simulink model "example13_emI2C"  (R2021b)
settings: Solver=FixedStepAuto  StartTime=0  StopTime=inf  FixedStep=0.5  RelTol=1e-3  EnableMultiTasking=on
undefined symbols (not defined in the file or in its folder): based, Big, bits, bus, classic, dsPic33, Endian, I2C, MCC, Microchip, PIC24
libraries: emSPII2CLib x6, embeddedCreatorLib x6, emMBSlaveLib x1

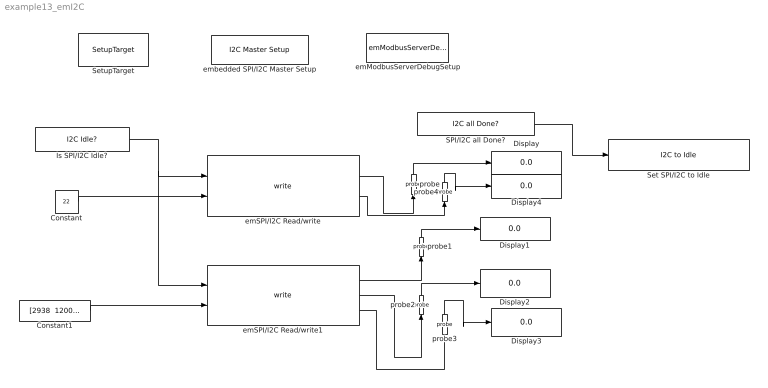
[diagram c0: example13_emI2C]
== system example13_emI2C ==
  Constant : Constant  Value=22  OutDataTypeStr=int8
  Constant1 : Constant  Value="[2938  12000]"  OutDataTypeStr=int16
  Display{,1..4} (5 alike) : Display
  Is SPI/I2C Idle? : emSPII2CLib/Is SPI//I2C Idle?  Tag=isSPI_I2C_Idle  c_DeviceNo=2  c_BusType=I2C bus  c_sampleTime=-1
  SPI/I2C all Done? : emSPII2CLib/SPI//I2C all Done?  c_DeviceNo=2  c_BusType=I2C bus  c_sampleTime=-1
  Set SPI/I2C to Idle : emSPII2CLib/Set SPI//I2C to Idle  Tag=setSPI_I2C2Idle  c_DeviceNo=2  c_BusType=I2C bus
  SetupTarget : embeddedCreatorLib/SetupTarget  Tag=SetupTarget  Priority=0  c_platform=Microchip PIC24/dsPic33 based on MCC classic  c_debug=on
  emModbusServerDebugSetup : emMBSlaveLib/emModbusServerDebugSetup  Tag=emModbusSlaveSetup  c_objID=0  c_uartNo=2  c_baudrate=19200  c_serverID=1  c_baudrate4PC=19200  c_forceLongerSpace=on  c_holdingRegsQTY=0  c_minHoldingAddr=789  c_inputRegsQTY=0  c_minInputRegAddr=20  c_coilRegsQTY=0  c_minCoilAddr=30  c_discreteRegsQTY=0  c_minDiscreteAddr=40  c_enableDebug=on  c_breakpointMaxQTY=0  c_probeMaxWordQTY=100  c_emWaitQTY=0  g_COMPortNo=COM5  c_Name_method=By physical port name and bit number  c_PortName=B  c_BitNo=11  c_TxEnable485="\"LATBbits.LATB11\""  c_TxEnable485Polarity=on
  emSPI/I2C Read/write : emSPII2CLib/emSPI//I2C Read//write  Tag=emSPII2CWR  c_DeviceNo=2  c_BusType=I2C bus  c_SeqNo=Seq0  c_How_to_specifyCS=By physical port name and bit number  c_PortName=D  c_BitNumber=8  c_CSAccessName="\"LATDbits.LATD8\""  c_CS_Polarity=on  c_SPI_dummyData=ALL bits Logic low  c_I2CAddress=1  c_Endian=Big-Endian  c_WriteDataType=[int8]  c_InputDataQty=[1]  c_InputType=[2]  c_OutputDataQty=[]  c_OutputType=[]
  emSPI/I2C Read/write1 : emSPII2CLib/emSPI//I2C Read//write  Tag=emSPII2CWR  c_DeviceNo=2  c_BusType=I2C bus  c_SeqNo=Seq1  c_How_to_specifyCS=By physical port name and bit number  c_PortName=D  c_BitNumber=8  c_CSAccessName="\"LATDbits.LATD8\""  c_CS_Polarity=on  c_SPI_dummyData=ALL bits Logic low  c_I2CAddress=1  c_Endian=Big-Endian  c_ReadDataType=int8  c_WriteDataType=[int16*2]  c_InputDataQty=[2]  c_InputType=[4]  c_OutputDataQty=[1]  c_OutputType=[2]
  embedded SPI/I2C Master Setup : emSPII2CLib/embedded SPI//I2C Master Setup  Tag=emSPI_I2CMaster  c_DeviceNo=2  c_BusType=I2C bus  c_SPI_Data_width=8 bits  c_SPI_ByteQty=8  c_MAX_SeqQTY=4  c_I2C_MaxBytes4W=6  c_I2C_MaxBytes4R=6
  probe : embeddedCreatorLib/probe  Tag=emProbe  c_ObjID=3  c_serverID=1  c_UartNo=1  c_StartAddr=5  c_ConstantDataSource=off
  probe1 : embeddedCreatorLib/probe  Tag=emProbe  c_ObjID=0  c_serverID=1  c_UartNo=1  c_StartAddr=2  c_ConstantDataSource=off
  probe2 : embeddedCreatorLib/probe  Tag=emProbe  c_ObjID=1  c_serverID=1  c_UartNo=1  c_StartAddr=3  c_ConstantDataSource=off
  probe3 : embeddedCreatorLib/probe  Tag=emProbe  c_ObjID=2  c_serverID=1  c_UartNo=1  c_StartAddr=4  c_ConstantDataSource=off
  probe4 : embeddedCreatorLib/probe  Tag=emProbe  c_ObjID=4  c_serverID=1  c_UartNo=1  c_StartAddr=6  c_ConstantDataSource=off
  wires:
  Is SPI/I2C Idle?/1 -> emSPI/I2C Read/write1/1, emSPI/I2C Read/write/1
  SPI/I2C all Done?/1 -> Set SPI/I2C to Idle/1
  Constant/1 -> emSPI/I2C Read/write/2
  Constant1/1 -> emSPI/I2C Read/write1/2
  emSPI/I2C Read/write/1 -> probe/1
  probe/1 -> Display/1
  emSPI/I2C Read/write1/1 -> probe1/1
  probe1/1 -> Display1/1
  emSPI/I2C Read/write1/2 -> probe2/1
  probe2/1 -> Display2/1
  emSPI/I2C Read/write1/3 -> probe3/1
  probe3/1 -> Display3/1
  emSPI/I2C Read/write/2 -> probe4/1
  probe4/1 -> Display4/1
